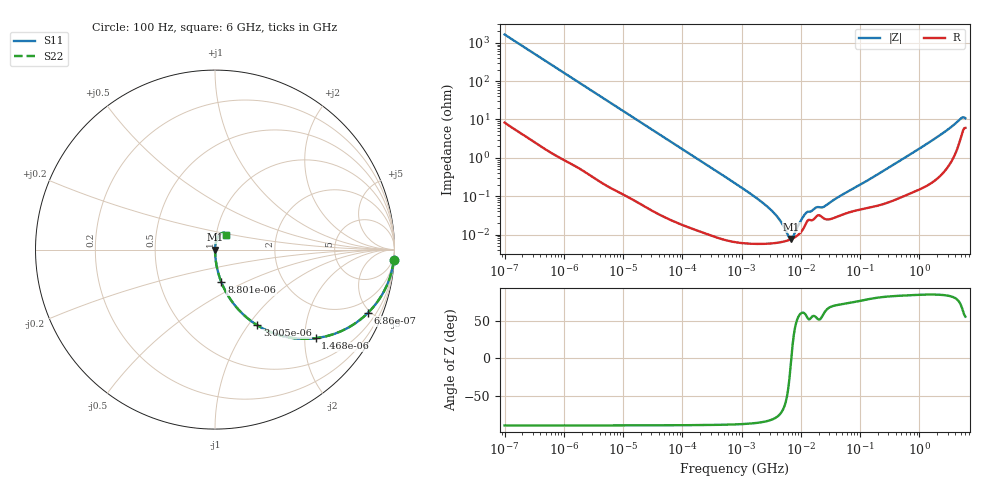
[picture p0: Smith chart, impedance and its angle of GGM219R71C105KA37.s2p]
!Murata Part Number: GGM219R71C105KA37
!These Parameters are Measured in Series Mode Connection
!Data Generated on Jun 19, 2026
!  o--ll--o
!Port1  Port2
!  o------o
!Operation Temp=25[degC], DC Bias Voltage=0[V]
!Freq. Start=100[Hz] Stop=6[GHz] 401[Steps]
# Hz S RI R 50
!Freq.(Hz) S11(Real) S11(Imag) S21(Real) S21(Imag) S12(Real) S12(Imag) S22(Real) S22(Imag)
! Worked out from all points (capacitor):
!   401 points, 100 Hz to 6 GHz, reference 50 ohm
!   read as one part in series: C = 967 nF near 109 Hz
!   lowest |Z| = 7.63 mohm at 6.949 MHz (marker M1)
!   series resonance near 6.91 MHz, so ESL is about 550 pH
!   S11 on the Smith chart (normalised r, x): 100 Hz: 1, -33; 686 Hz: 1.02, -4.82; 1.468 kHz: 1.01, -2.26; 3.005 kHz: 1.01, -1.11; 8.801 kHz: 1.00, -0.38; 6 GHz: 1.12, +0.18
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100  0.996 -0.0606  0.00399 0.0606  0.00399 0.0606  0.996 -0.0606
335  0.9595 -0.1946  0.0405 0.1946  0.0405 0.1946  0.9595 -0.1946
686  0.8519 -0.3527  0.1481 0.3527  0.1481 0.3527  0.8519 -0.3527
1468  0.56 -0.4936  0.44 0.4936  0.44 0.4936  0.56 -0.4936
2008  0.4062 -0.4882  0.5938 0.4882  0.5938 0.4882  0.4062 -0.4882
3005  0.2355 -0.4214  0.7645 0.4214  0.7645 0.4214  0.2355 -0.4214
4918  0.1042 -0.3026  0.8958 0.3026  0.8958 0.3026  0.1042 -0.3026
8801  0.0358 -0.1825  0.9642 0.1825  0.9642 0.1825  0.0358 -0.1825
40335  0.00206 -0.0415  0.9979 0.0415  0.9979 0.0415  0.00206 -0.0415
774597  6.8e-05 -0.00217  0.9999 0.00217  0.9999 0.00217  6.8e-05 -0.00217
2837864  5.81e-05 -0.000501  0.9999 0.000501  0.9999 0.000501  5.81e-05 -0.000501
4246196  6.18e-05 -0.000252  0.9999 0.000252  0.9999 0.000252  6.18e-05 -0.000252
5809218  6.89e-05 -8.76e-05  0.9999 8.76e-05  0.9999 8.76e-05  6.89e-05 -8.76e-05
6948629  7.62e-05 2.9e-06  0.9999 -2.9e-06  0.9999 -2.9e-06  7.62e-05 2.9e-06
7947587  8.49e-05 7.2e-05  0.9999 -7.2e-05  0.9999 -7.2e-05  8.49e-05 7.2e-05
1.189169e7  0.000178 0.000299  0.9998 -0.000299  0.9998 -0.000299  0.000178 0.000299
1.555665e7  0.000236 0.000349  0.9998 -0.000349  0.9998 -0.000349  0.000236 0.000349
2.545746e7  0.000255 0.000486  0.9997 -0.000486  0.9997 -0.000486  0.000255 0.000486
3.124326e8  0.000733 0.00564  0.9993 -0.00564  0.9993 -0.00564  0.000733 0.00564
1.95892e9  0.0039 0.0336  0.9961 -0.0336  0.9961 -0.0336  0.0039 0.0336
5.016141e9  0.041 0.0929  0.959 -0.0929  0.959 -0.0929  0.041 0.0929
6e9  0.0636 0.0787  0.9364 -0.0787  0.9364 -0.0787  0.0636 0.0787
